(* Logix 5000 AddOnInstructionDefinition export AKD_Command_Control_Word; software revision 19.01 *)

TYPE AKD_Status :   // All connections to the drive ethernet module are established and data is successfully transferring.
STRUCT
   Profile_In_Progress : BOOL;   // Profile Move In Progress
   Block_In_Execution : BOOL;   // Block In Execution
   On_Target_Position : BOOL;   // On Target Position (1=Current Position Equals Last Target Position)
   General_Fault : BOOL;   // General Fault
   Current_Direction : BOOL;   // Current Motor Direction (0=Reverse, 1=Forward)
   Home_Level : BOOL;   // Level of Home Input
   Reg_Level : BOOL;   // Level of Registration Input
   Enable : BOOL;   // State of Enable Output
   Fault_Input_Fault : BOOL;   // Fault Input Active
   Fwd_Limit : BOOL;   // Forward Input Active
   Rev_Limit : BOOL;   // Reverse Input Active
   Positive_Limit : BOOL;   // Positive Software Limit Exceeded
   Negative_Limit : BOOL;   // Negative Software Limit Exceeded
   FE_Fault : BOOL;   // Following Error Fault
   Block_Fault : BOOL;   // Block Execution Fault
   Load_Complete : BOOL;   // Command Message Successfully Loaded
END_STRUCT
END_TYPE

TYPE AKD_Control :   // Send Explicit Message
STRUCT
   Load_Data_Start_Profile : BOOL;   // Load Command Data / Start Profile Move
   Start_Block : BOOL;   // Execute Command block or block chain
   Incremental : BOOL;   // Incremental Position (0=Absolute, 1=Incremental)
   Direction : BOOL;   // Direction in Velocity Mode (0=Reverse, 1=Forward)
   Smooth_Stop : BOOL;   // Smooth / Controlled Stop w/ Deceleration
   Hard_Stop : BOOL;   // Hard / Immediate Stop
   Reg_Arm : BOOL;   // Arm the Registration Input
   Enable : BOOL;   // Enable Output
END_STRUCT
END_TYPE

TYPE AKD_Axis :   // Axis Data:
STRUCT
   Control : AKD_Control;   // Control bits to send to the drive
   Status : AKD_Status;   // Status bits received from the drive
   Input : AB:ETHERNET_MODULE_SINT_64Bytes:I:0;   // Data from the drive
   Output : AB:ETHERNET_MODULE_SINT_64Bytes:O:0;   // Data to the drive
   ResponseMsgType : SINT;   // Response type contained in latest IO response from drive. Used to check for errors
   CommandTimeout : INT;   // Time to allow for command response from drive. Dependent on scan rate and communicaiton rate
   PositionFeedback : DINT;   // Actual Position Value
   VelocityFeedback : DINT;   // Actual Velocity Value
END_STRUCT
END_TYPE

ADD_ON_INSTRUCTION AKD_Command_Control_Word   (* revision 1.0 *)
VAR_IN_OUT
   Axis : AKD_Axis; {required}
END_VAR
VAR_OUTPUT
   Load_Start : BOOL; {access Read Only, visible}
   Start_Block : BOOL; {access Read Only, visible}
   Relative : BOOL; {access Read Only, visible}
   Direction : BOOL; {access Read Only, visible}
   Smooth_Stop : BOOL; {access Read Only, visible}
   Hard_Stop : BOOL; {access Read Only, visible}
   Reserved_Bit_6 : BOOL; {access Read Only, visible}
   Enable : BOOL; {access Read Only, visible}
END_VAR

ROUTINE Logic   (* ladder *)
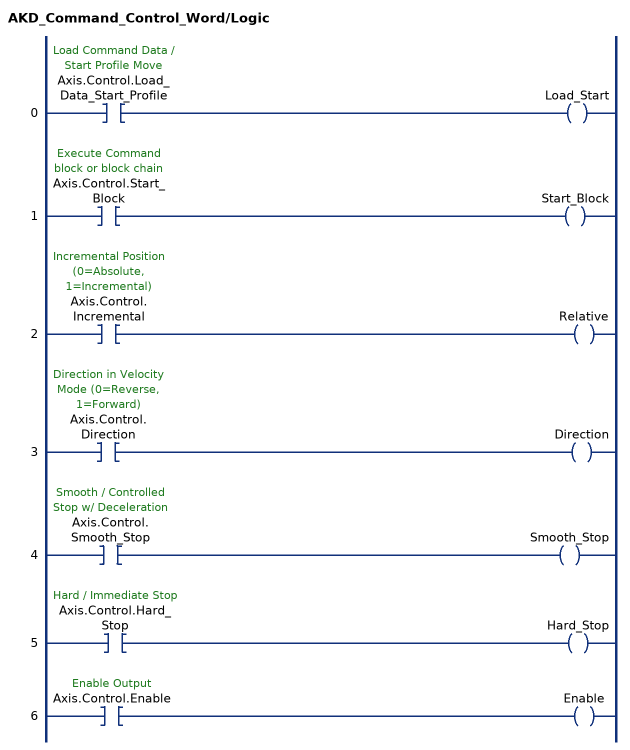
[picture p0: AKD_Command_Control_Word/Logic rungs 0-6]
   0: XIC(Axis.Control.Load_Data_Start_Profile)OTE(Load_Start);
   1: XIC(Axis.Control.Start_Block)OTE(Start_Block);
   2: XIC(Axis.Control.Incremental)OTE(Relative);
   3: XIC(Axis.Control.Direction)OTE(Direction);
   4: XIC(Axis.Control.Smooth_Stop)OTE(Smooth_Stop);
   5: XIC(Axis.Control.Hard_Stop)OTE(Hard_Stop);
   6: XIC(Axis.Control.Enable)OTE(Enable);
END_ROUTINE
END_ADD_ON_INSTRUCTION
